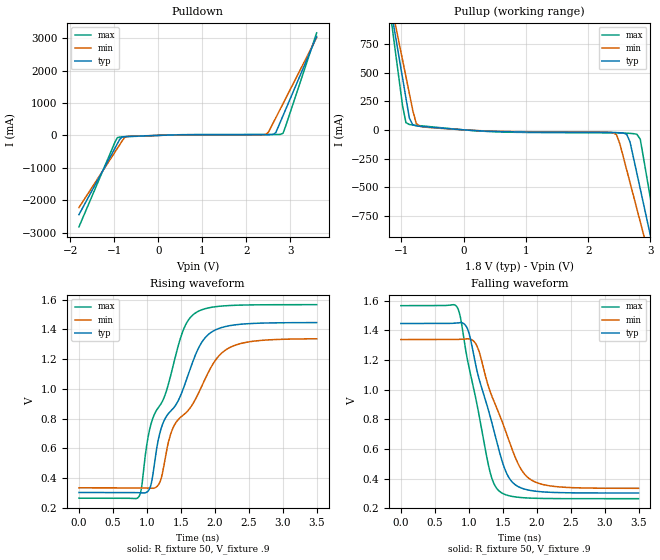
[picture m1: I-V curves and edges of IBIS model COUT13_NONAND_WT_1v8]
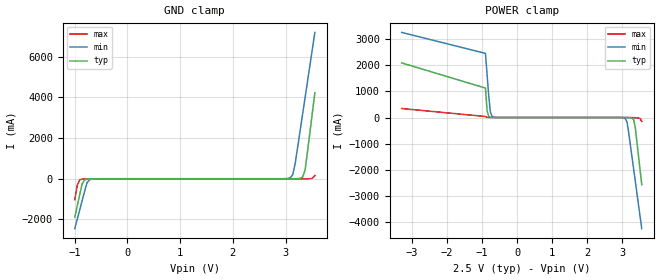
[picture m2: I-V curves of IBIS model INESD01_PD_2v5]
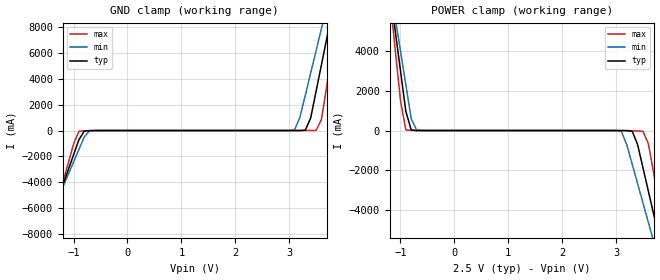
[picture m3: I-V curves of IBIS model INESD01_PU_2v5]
|   This file is an IBIS representation of the   |
|   Integrated Devices Technology, Inc.   |
|   ICS81006   |
|   VCXO-TO-6 LVCMOS OUTPUTS   |
[IBIS Ver]   4.1
[File name]   81006.ibs
[File Rev]   1.0
[Date]   28 Apr 2009 | Last modified
|   Oct 06 2004 | Generated
[Source]   Originated at Integrated Devices Technology, Inc.
[Disclaimer]
IDT hereby grants the user of this IBIS model a non-exclusive,
nontransferable license to use this IBIS model under the following terms.
Before using this IBIS model, the user should read this license.
If the user does not accept these terms,  the IBIS model should be
returned to IDT within 30 days.
   The user is granted this license only to use the IBIS model and
is not granted rights to sell, load, rent, lease or license the IBIS
model in whole or in part, or in modified form to anyone other than
user. User may modify the IBIS model to suit its specific
applications but rights to derivative works and such modifications
shall belong to IDT.
   This IBIS model is provided on an "AS IS" basis and IDT makes
absolutely no warranty with respect to the information contained
herein. IDT DISCLAIMS AND CUSTOMER WAIVES ALL WARRANTIES, EXPRESS
OR IMPLIED, INCLUDING WARRANTIES OF MERCHANTABILITY OR FITNESS FOR
A PARTICULAR PURPOSE. The entire risk as to quality and performance
is with the Customer. ACCORDINGLY, IN NO EVENT SHALL THE COMPANY BE
LIABLE FOR ANY DAMAGES, WHETHER IN CONTRACT OR TORT,INCLUDING ANY
LOST PROFITS OR OTHER INCIDENTAL, CONSEQUENTIAL, EXEMPLARY, OR
PUNITIVE DAMAGES ARISING OUT OF THE USE OR APPLICATION OF THE IBIS
model provided in this package. Further, IDT reserves the right to
make changes without notice to any product herein to improve
reliability, function, or design. IDT does not convey any license
under patent rights or any other intellectual property rights,
including those of third parties.
   IDT is not obligated to provide maintenance or support
for the licensed IBIS model.
[Copyright]   Copyright 2004 by Integrated Devices Technology, Inc.
[Component]   ICS83905AK
[Manufacturer] Integrated Devices Technology, Inc.
[Package]
|VFQFN 20   typ   min   max
R_pkg   72.4655m   58.886m   86.045m
L_pkg   1.47175nH   1.11650nH   1.77850n
C_pkg   0.07747pF   0.07444pF   0.08050pF
[Pin] signal_name   model_name   R_pin   L_pin   C_pin
1   XTAL_IN   NC   86.0450m   1.7785n   0.08050p
2   XTAL_OUT   NC   72.4655m   1.4475n   0.07747p
3   VDD   POWER   58.8860m   1.1165n   0.07444p
4   VC   NC   72.4655m   1.4475n   0.07747p
5   DIV_SEL_Q5 INESD01_PD   86.0450m   1.7785n   0.08050p
6   OE1   INESD01_PU   86.0450m   1.7785n   0.08050p
7   GND   GND   72.4655m   1.4475n   0.07747p
8   Q5   COUT13_NONAND_WT   58.8860m   1.1165n   0.07444p
9   VDDO   POWER   72.4655m   1.4475n   0.07747p
10  Q4   COUT13_NONAND_WT   86.0450m   1.7785n   0.08050p
11  GND   GND   86.0450m   1.7785n   0.08050p
12  Q3   COUT13_NONAND_WT   72.4655m   1.4475n   0.07747p
13  VDDO   POWER   58.8860m   1.1165n   0.07444p
14  Q2   COUT13_NONAND_WT   72.4655m   1.4475n   0.07747p
15  GND   GND   86.0450m   1.7785n   0.08050p
16  Q1   COUT13_NONAND_WT   86.0450m   1.7785n   0.08050p
17  VDDO   POWER   72.4655m   1.4475n   0.07747p
18  Q0   COUT13_NONAND_WT   58.8860m   1.1165n   0.07444p
19  GND   GND   72.4655m   1.4475n   0.07747p
20  OE0   INESD01_PU   86.0450m   1.7785n   0.08050p
[Model Selector] INESD01_PD
INESD01_PD_2v5  Buffer selection for 2v5
INESD01_PD_3v3  Buffer selection for 3v3
[Model Selector] INESD01_PU
INESD01_PU_2v5  Buffer selection for 2v5
INESD01_PU_3v3  Buffer selection for 3v3
[Model Selector] COUT13_NONAND_WT
COUT13_NONAND_WT_1v8  Buffer selection for 1v8
COUT13_NONAND_WT_2v5  Buffer selection for 2v5
COUT13_NONAND_WT_3v3  Buffer selection for 3v3
| Models and submodels in the file (7): COUT13_NONAND_WT_1v8 (Output), INESD01_PD_2v5 (Input), INESD01_PU_2v5 (Input), COUT13_NONAND_WT_2v5 (Output), INESD01_PD_3v3 (Input), INESD01_PU_3v3 (Input), COUT13_NONAND_WT_3v3 (Output)
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[Model] COUT13_NONAND_WT_1v8
Model_type   Output
Polarity   Non-Inverting
|   typ   min   max
C_comp   2pF   1.5pF   2.5pF
Vmeas = .9
Rref = 50
Cref = 0
Vref = .9
|   typ   min   max
[Voltage range]   1.8V   1.710V   1.890V
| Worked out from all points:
|   slope of the pulldown table from 0 to 0.27 V, typ, clamps not added: 24.7 ohm
|   slope of the pullup table from 0 to 0.27 V, typ, clamps not added: 30.7 ohm
|   rising waveform, R_fixture 50, V_fixture .9: 20-80 % time 583ps typ, 664ps min, 502ps max; typ from 0.303 V to 1.45 V
|   falling waveform, R_fixture 50, V_fixture .9: 20-80 % time 402ps typ, 471ps min, 333ps max; typ from 1.45 V to 0.303 V
[Pulldown]
|Voltage   I (typ)   I (min)   I (max)
-1.8V     -2.442A    -2.223A    -2.818A
-981.8mV  -392.3mA   -512.3mA   -207.3mA
-927.3mV  -255.5mA   -398.3mA   -69.39mA
-818.2mV  -48.44mA   -170.3mA   -45.64mA
-763.6mV  -37.2mA    -65.77mA   -42.22mA
-654.5mV  -30.39mA   -27.15mA   -35.88mA
2.455V    23.11mA    35.96mA    27.64mA
2.509V    23.53mA    110.5mA    27.69mA
2.618V    32.43mA    399.5mA    27.88mA
2.673V    89.99mA    544.3mA    28.15mA
2.836V    608.7mA    979.1mA    66.58mA
3.6V      3.051A     3.016A     3.161A
[Pullup]
|Voltage   I (typ)   I (min)   I (max)
-1.8V     3.082A     2.802A     3.565A
-1.145V   977.3mA    1.047A     881.2mA
-981.8mV  451.6mA    609mA      210.5mA
-872.7mV  103.4mA    317mA      46.54mA
-763.6mV  34.53mA    57.78mA    39.56mA
-654.5mV  28.37mA    25.5mA     33.72mA
2.4V      -23.05mA   -25.3mA    -26.17mA
2.618V    -37.89mA   -348.5mA   -29.19mA
2.782V    -378.8mA   -688.4mA   -38.24mA
3V        -923mA     -1.142A    -598.7mA
3.109V    -1.195A    -1.37A     -946.1mA
3.6V      -2.422A    -2.393A    -2.51A
[Ramp]
|   typ   min   max
dV/dt_r   0.917/0.749n   0.804/0.862n   1.043/0.638n
dV/dt_f   0.918/0.549n   0.806/0.65n   1.046/0.449n
R_load =   50.0000
[Rising Waveform]
R_fixture = 50
V_fixture = .9   |Vcc_typ
V_fixture_min = .855 |Vcc_min
V_fixture_max = .945 |Vcc_max
C_fixture = 0.0p
| Time   typ   min   max
0s        302.6mV    334.1mV    264.3mV
882.9ps   300.8mV    334.1mV    275.8mV
1.069ns   372.7mV    330.3mV    776.9mV
1.219ns   747.8mV    414.6mV    908.8mV
1.38ns    865.1mV    733.6mV    1.146V
1.535ns   1.001V     823.4mV    1.395V
1.685ns   1.195V     906.4mV    1.501V
1.888ns   1.359V     1.097V     1.542V
2.214ns   1.424V     1.277V     1.56V
3.497ns   1.445V     1.336V     1.566V
[Falling Waveform]
R_fixture = 50
V_fixture = .9   |Vcc_typ
V_fixture_min = .855 |Vcc_min
V_fixture_max = .945 |Vcc_max
C_fixture = 0.0p
| Time   typ   min   max
0s        1.446V     1.337V     1.566V
833.8ps   1.45V      1.338V     1.551V
981ps     1.408V     1.342V     1.197V
1.107ns   1.152V     1.305V     929.3mV
1.314ns   819.3mV    985.7mV    440.7mV
1.454ns   573.6mV    826.6mV    312.8mV
1.633ns   379.4mV    602.2mV    280mV
1.78ns    334.8mV    454.7mV    271.5mV
1.944ns   317mV      383.7mV    267.5mV
3.497ns   302.6mV    334.2mV    264.4mV
[Model] INESD01_PD_2v5
Model_type   Input
Polarity   Non-Inverting
Vinl = 0.8V
Vinh = 2.0V
|   typ   min   max
C_comp   2pF   1.5pF   2.5pF
|   typ   min   max
[Voltage range]  2.5V   2.375V   2.625V
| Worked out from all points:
|   GND clamp passes 1 mA (typ) near -0.55 V on its own axis
|   POWER clamp passes 1 mA (typ) near -0.68 V on its own axis
[GND_clamp]
|Voltage I(typ)   I(min)   I(max)
-1V       -1.886A    -2.451A    -1.028A
-953.5mV  -1.338A    -1.994A    -328mA
-907mV    -789.6mA   -1.537A    -53.04mA
-860.5mV  -251.4mA   -1.081A    -21.51mA
-767.5mV  -17.28mA   -198.8mA   -10.01mA
-674.5mV  -5.28mA    -15.38mA   -3.684mA
3.092V    224.5uA    49.06mA    51.52uA
3.139V    500.8uA    208.3mA    52.98uA
3.185V    1.252mA    774.6mA    56.66uA
3.325V    81.55mA    3.177A     200uA
3.371V    416.9mA    3.978A     464.6uA
3.557V    4.225A     7.185A     159.2mA
[POWER_clamp]
|Voltage   I(typ)   I(min)   I(max)
-3.3V     2.083A     3.246A     343.1mA
-907mV    1.122A     2.445A     37.78mA
-860.5mV  267.5mA    1.644A     5.973mA
-814mV    47.03mA    844mA      1.727mA
-767.5mV  9.66mA     215.3mA    677uA
-674.5mV  960.6uA    12.66mA    131.4uA
3.092V    -1.849mA   -49.09mA   -51.51uA
3.139V    -3.491mA   -186mA     -159.7uA
3.325V    -84.03mA   -1.955A    -5.102mA
3.371V    -365.4mA   -2.411A    -8.31mA
3.51V     -2.01A     -3.782A    -35.44mA
3.557V    -2.558A    -4.239A    -152.3mA
[Model] INESD01_PU_2v5
Model_type   Input
Polarity   Non-Inverting
Vinl = 1.4V
Vinh = 1.85V
|   typ   min   max
C_comp   2pF   1.5pF   2.5pF
|   typ   min   max
[Voltage range]  2.5V   2.375V   2.625V
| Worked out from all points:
|   GND clamp passes 1 mA (typ) near -0.54 V on its own axis
|   POWER clamp passes 1 mA (typ) near -0.66 V on its own axis
[GND_clamp]
|Voltage   I(typ)   I(min)   I(max)
-2.5V     -19.6A     -17.18A    -23.67A
-1.6V     -8.969A    -8.332A    -10.1A
-1.5V     -7.788A    -7.349A    -8.588A
-900mV    -707.1mA   -1.46A     -57.43mA
-700mV    -7.027mA   -24.05mA   -13.28mA
3.1V      199.2uA    53.94mA    11.78uA
3.3V      28.4mA     2.748A     652.4uA
3.5V      3.045A     6.192A     15.72mA
3.6V      5.115A     7.914A     872.4mA
3.7V      7.185A     9.638A     3.52A
3.9V      11.33A     13.09A     8.818A
5V        34.14A     32.07A     37.99A
[POWER_clamp]
|Voltage   I(typ)   I(min)   I(max)
-1.5V     9.257A     9.207A     9.48A
-1.2V     7.185A     7.484A     6.83A
-1.1V     5.115A     5.761A     4.182A
-900mV    976.9mA    2.318A     34.23mA
-700mV    1.582mA    24.31mA    1.044mA
3.1V      -2.107mA   -51.03mA   -534.5uA
3.3V      -35.62mA   -1.705A    -10.86mA
3.5V      -1.886A    -3.666A    -39.41mA
3.6V      -3.066A    -4.647A    -666.9mA
3.8V      -5.426A    -6.612A    -3.684A
3.9V      -6.607A    -7.595A    -5.193A
5V        -19.6A     -18.41A    -21.79A
